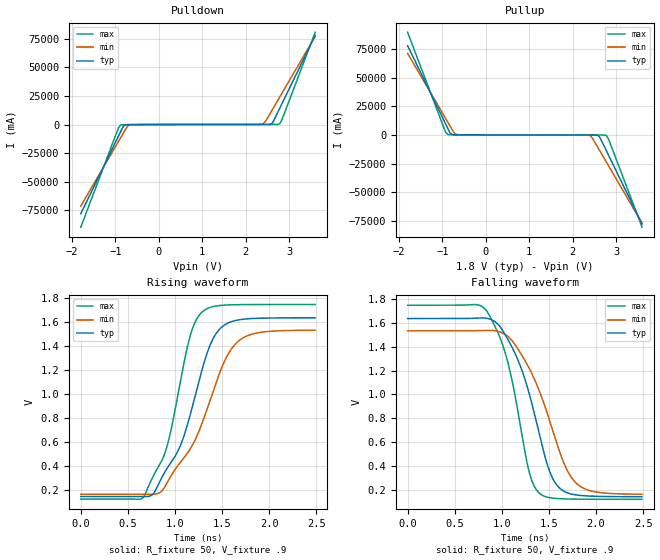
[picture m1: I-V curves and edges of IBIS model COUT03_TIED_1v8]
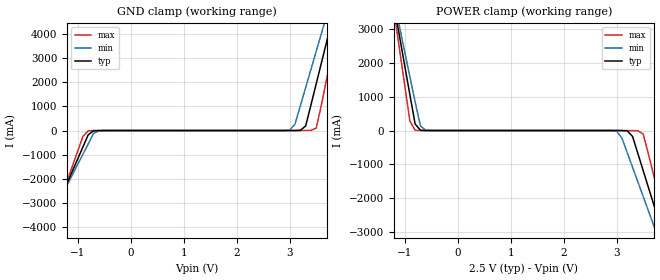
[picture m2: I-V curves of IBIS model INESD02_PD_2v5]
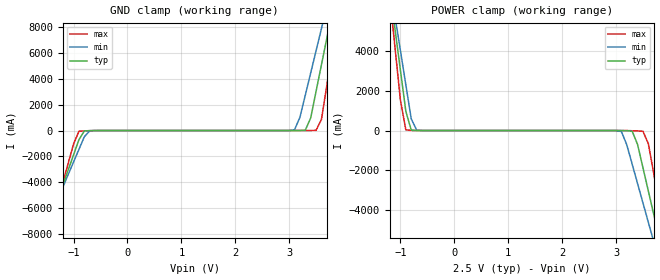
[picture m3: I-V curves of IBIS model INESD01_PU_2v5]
|   This file is an IBIS representation of the   |
|   Integrated Devices Technology, Inc.   |
|   ICS87016   |
|   LOW SKEW, 1-TO-16 LVCMOS/LVTTL CLOCK GENERATOR   |
[IBIS Ver]   4.1
[File name]   87016.ibs
[File Rev]   1.0
[Date]   13 Apr 2009 | Last modified
|   Jan 09 2003 | Generated
[Source]   Originated at Integrated Devices Technology, Inc.
[Disclaimer]
IDT hereby grants the user of this IBIS model a non-exclusive,
nontransferable license to use this IBIS model under the following terms.
Before using this IBIS model, the user should read this license.
If the user does not accept these terms,  the IBIS model should be
returned to IDT within 30 days.
   The user is granted this license only to use the IBIS model and
is not granted rights to sell, load, rent, lease or license the IBIS
model in whole or in part, or in modified form to anyone other than
user. User may modify the IBIS model to suit its specific
applications but rights to derivative works and such modifications
shall belong to IDT.
   This IBIS model is provided on an "AS IS" basis and IDT makes
absolutely no warranty with respect to the information contained
herein. IDT DISCLAIMS AND CUSTOMER WAIVES ALL WARRANTIES, EXPRESS
OR IMPLIED, INCLUDING WARRANTIES OF MERCHANTABILITY OR FITNESS FOR
A PARTICULAR PURPOSE. The entire risk as to quality and performance
is with the Customer. ACCORDINGLY, IN NO EVENT SHALL THE COMPANY BE
LIABLE FOR ANY DAMAGES, WHETHER IN CONTRACT OR TORT,INCLUDING ANY
LOST PROFITS OR OTHER INCIDENTAL, CONSEQUENTIAL, EXEMPLARY, OR
PUNITIVE DAMAGES ARISING OUT OF THE USE OR APPLICATION OF THE IBIS
model provided in this package. Further, IDT reserves the right to
make changes without notice to any product herein to improve
reliability, function, or design. IDT does not convey any license
under patent rights or any other intellectual property rights,
including those of third parties.
   IDT is not obligated to provide maintenance or support
for the licensed IBIS model.
[Copyright]   Copyright 2003 by Integrated Devices Technology, Inc.
[Component]   ICS87016
[Manufacturer] Integrated Devices Technology, Inc.
[Package]
|LQFP48
|lead + wire   typ   min   max
R_pkg   220.4m   212.5m   238m
L_pkg   1.841nH   1.708nH   1.974n
C_pkg   0.316pF   0.2907pF   0.33pF
[Pin] signal_name   model_name  R_pin   L_pin   C_pin
1   VDD   POWER   238m   1.974n   0.338p
2   CLK0   INESD02_PD   225m   1.831n   0.330p
3   DIV_SELA   INESD01_PU   220m   1.781n   0.323p
4   DIV_SELB   INESD01_PU   214m   1.732n   0.312p
5   DIV_SELC   INESD01_PU   214m   1.709n   0.305p
6   DIV_SELD   INESD01_PU   213m   1.708n   0.291p
7   CLK_ENA   INESD01_PU   213m   1.708n   0.291p
8   CLK_ENB   INESD01_PU   214m   1.709n   0.305p
9   CLK_ENC   INESD01_PU   214m   1.732n   0.312p
10   CLK_END   INESD01_PU   220m   1.781n   0.323p
11   nMR/OE   INESD01_PU   225m   1.831n   0.330p
12   GND   GND   238m   1.974n   0.338p
13   QD3   COUT03_TIED  238m   1.974n   0.338p
14   VDDOD   POWER   225m   1.831n   0.330p
15   QD2   COUT03_TIED  220m   1.781n   0.323p
16   GND   GND   214m   1.732n   0.312p
17   QD1   COUT03_TIED  214m   1.709n   0.305p
18   VDDOD   POWER   213m   1.708n   0.291p
19   QD0   COUT03_TIED  213m   1.708n   0.291p
20   GND   GND   214m   1.709n   0.305p
21   QC3   COUT03_TIED  214m   1.732n   0.312p
22   VDDOC   POWER   220m   1.781n   0.323p
23   QC2   COUT03_TIED  225m   1.831n   0.330p
24   GND   GND   238m   1.974n   0.338p
25   QC1   COUT03_TIED  238m   1.974n   0.338p
26   VDDOC   POWER   225m   1.831n   0.330p
27   QC0   COUT03_TIED  220m   1.781n   0.323p
28   GND   GND   214m   1.732n   0.312p
29   QB3   COUT03_TIED  214m   1.709n   0.305p
30   VDDOB   POWER   213m   1.708n   0.291p
31   QB2   COUT03_TIED  213m   1.708n   0.291p
32   GND   GND   214m   1.709n   0.305p
33   QB1   COUT03_TIED  214m   1.732n   0.312p
34   VDDOB   POWER   220m   1.781n   0.323p
35   QB0   COUT03_TIED  225m   1.831n   0.330p
36   GND   GND   238m   1.974n   0.338p
37   QA3   COUT03_TIED  238m   1.974n   0.338p
38   VDDOA   POWER   225m   1.831n   0.330p
39   QA2   COUT03_TIED  220m   1.781n   0.323p
40   GND   GND   214m   1.732n   0.312p
41   QA1   COUT03_TIED  214m   1.709n   0.305p
42   VDDOA   POWER   213m   1.708n   0.291p
43   QA0   COUT03_TIED  213m   1.708n   0.291p
44   GND   GND   214m   1.709n   0.305p
45   CLK_SEL   INESD01_PD   214m   1.732n   0.312p
46   nCLK1   INESD01_PU   220m   1.781n   0.323p
47   CLK1   INESD01_PD   225m   1.831n   0.330p
48   VDD   POWER   238m   1.974n   0.338p
[Diff Pin]  inv_pin  vdiff tdelay_typ tdelay_min  tdelay_max
47   46   0.15   0   0   0
[Model Selector] INESD02_PD
INESD02_PD_2v5  Buffer selection for 2v5
INESD02_PD_3v3  Buffer selection for 3v3
[Model Selector] INESD01_PU
INESD01_PU_2v5  Buffer selection for 2v5
INESD01_PU_3v3  Buffer selection for 3v3
[Model Selector] COUT03_TIED
COUT03_TIED_1v8  Buffer selection for 1v8
COUT03_TIED_2v5  Buffer selection for 2v5
COUT03_TIED_3v3  Buffer selection for 3v3
[Model Selector] INESD01_PD
INESD01_PD_2v5  Buffer selection for 2v5
INESD01_PD_3v3  Buffer selection for 3v3
| Models and submodels in the file (9): COUT03_TIED_1v8 (Output), INESD02_PD_2v5 (Input), INESD01_PU_2v5 (Input), COUT03_TIED_2v5 (Output), INESD01_PD_2v5 (Input), INESD02_PD_3v3 (Input), INESD01_PU_3v3 (Input), COUT03_TIED_3v3 (Output), INESD01_PD_3v3 (Input)
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[Model] COUT03_TIED_1v8
Model_type   Output
Polarity   Non-Inverting
Vmeas = .9
Rref = 50
Cref = 0
Vref = .9
|   typ   min   max
C_comp   2pF   1.5pF   2.5pF
|   typ   min   max
[Voltage range]  1.8V   1.710V   1.890V
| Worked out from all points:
|   slope of the pulldown table from 0 to 0.27 V, typ, clamps not added: 10.3 ohm
|   slope of the pullup table from 0 to 0.27 V, typ, clamps not added: 11.9 ohm
|   rising waveform, R_fixture 50, V_fixture .9: 20-80 % time 370ps typ, 453ps min, 278ps max; typ from 0.143 V to 1.64 V
|   falling waveform, R_fixture 50, V_fixture .9: 20-80 % time 327ps typ, 389ps min, 257ps max; typ from 1.64 V to 0.143 V
[pulldown]
|Voltage   I (typ)   I (min)   I (max)
-1.8V     -77.88A    -71.2A     -89.55A
-927.3mV  -9.821A    -14.52A    -2.535A
-872.7mV  -5.567A    -10.98A    -279.7mA
-818.2mV  -1.447A    -7.441A    -119.4mA
-709.1mV  -98.56mA   -919.5mA   -92.65mA
-654.5mV  -74.81mA   -208.2mA   -85.34mA
2.4V      58.79mA    507.6mA    70.84mA
2.455V    61.02mA    2.637A     70.98mA
2.618V    1.414A     13.25A     71.57mA
2.782V    14.02A     23.86A     493.4mA
2.836V    18.27A     27.4A      4.385A
3.6V      77.78A     76.94A     80.46A
[pullup]
|Voltage   I (typ)   I (min)   I (max)
-1.8V     77.89A     71.2A      89.57A
-927.3mV  9.823A     14.53A     2.543A
-872.7mV  5.569A     10.98A     287mA
-818.2mV  1.45A      7.444A     126.9mA
-709.1mV  101.7mA    922.5mA    99.62mA
-654.5mV  77.73mA    211.3mA    91.37mA
2.4V      -60.59mA   -515mA     -72.08mA
2.455V    -64.65mA   -2.647A    -72.76mA
2.618V    -1.428A    -13.27A    -79.03mA
2.782V    -14.05A    -23.89A    -515mA
2.836V    -18.3A     -27.43A    -4.411A
3.6V      -77.85A    -77.01A    -80.54A
[Ramp]
|   typ   min   max
dV/dt_r   1.195/0.568n   1.097/0.672n   1.302/0.454n
dV/dt_f   1.198/0.499n   1.099/0.587n   1.305/0.4n
[Rising Waveform]
R_fixture = 50
V_fixture = .9
V_fixture_max = .945
V_fixture_min = .855
C_fixture = 0.0p
| Time   typ   min   max
0s        142.8mV    161.8mV    121.5mV
669.8ps   141.6mV    161.9mV    141.9mV
771.9ps   167.8mV    161.3mV    317mV
901.4ps   358.7mV    236.1mV    524.7mV
1.043ns   542.1mV    414.8mV    1.045V
1.17ns    851.2mV    551.4mV    1.508V
1.295ns   1.223V     771mV      1.689V
1.449ns   1.518V     1.122V     1.736V
1.678ns   1.619V     1.444V     1.746V
2.488ns   1.636V     1.533V     1.747V
[Falling Waveform]
R_fixture = 50
V_fixture = .9
V_fixture_max = .945
V_fixture_min = .855
C_fixture = 0.0p
| Time   typ   min   max
0s        1.636V     1.533V     1.747V
844.1ps   1.637V     1.538V     1.693V
1.021ns   1.52V      1.509V     1.386V
1.15ns    1.326V     1.405V     945.8mV
1.287ns   1.015V     1.223V     360mV
1.402ns   652.9mV    1.021V     170.3mV
1.559ns   269.5mV    650.9mV    130mV
1.673ns   183.5mV    397.7mV    124.9mV
1.783ns   159mV      262.2mV    123.1mV
2.488ns   143.1mV    163.6mV    121.5mV
[Model] INESD02_PD_2v5
Model_type   Input
Polarity   Non-Inverting
Vinl = 1.4V
Vinh = 1.85V
|   typ   min   max
C_comp   2pF   1.5pF   2.5pF
|   typ   min   max
[Voltage range]  2.5V   2.375V   2.625V
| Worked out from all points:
|   GND clamp passes 1 mA (typ) near -0.55 V on its own axis
|   POWER clamp passes 1 mA (typ) near -0.60 V on its own axis
[GND_clamp]
|Voltage I(typ)   I(min)   I(max)
-2.5V     -8.775A    -7.892A    -10.18A
-1.6V     -4.218A    -4.001A    -4.586A
-900mV    -678.5mA   -979.3mA   -237.6mA
-800mV    -173.9mA   -548.7mA   -10.83mA
-600mV    -1.629mA   -8.74mA    -911.1uA
3V        133.3uA    17.16mA    56.6uA
3.1V      660.9uA    273.5mA    60.87uA
3.3V      191.6mA    1.785A     327.9uA
3.5V      1.949A     3.298A     103.6mA
3.7V      3.723A     4.812A     2.189A
3.9V      5.498A     6.327A     4.369A
5V        15.27A     14.67A     16.38A
[POWER_clamp]
|Voltage   I(typ)   I(min)   I(max)
-2.5V     15.27A     13.72A     17.74A
-1.2V     3.723A     3.866A     3.551A
-1.1V     2.836A     3.109A     2.461A
-900mV    1.063A     1.596A     283.3mA
-800mV    191.6mA    840.1mA    6.189mA
-600mV    660.9uA    8.845mA    114.2uA
3V        -338.1uA   -16.36mA   -12.68uA
3.4V      -678.5mA   -1.518A    -7.183mA
3.5V      -1.183A    -1.95A     -99.52mA
3.7V      -2.195A    -2.813A    -1.324A
4V        -3.712A    -4.109A    -3.188A
5V        -8.775A    -8.432A    -9.404A
[Model] INESD01_PU_2v5
Model_type   Input
Polarity   Non-Inverting
Vinl = 1.4V
Vinh = 1.85V
|   typ   min   max
C_comp   2pF   1.5pF   2.5pF
|   typ   min   max
[Voltage range]  2.5V   2.375V   2.625V
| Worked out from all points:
|   GND clamp passes 1 mA (typ) near -0.54 V on its own axis
|   POWER clamp passes 1 mA (typ) near -0.66 V on its own axis
[GND_clamp]
|Voltage   I(typ)   I(min)   I(max)
-2.5V     -19.6A     -17.18A    -23.67A
-1.6V     -8.969A    -8.332A    -10.1A
-1.5V     -7.788A    -7.349A    -8.588A
-900mV    -707.1mA   -1.46A     -57.43mA
-700mV    -7.027mA   -24.05mA   -13.28mA
3.1V      199.2uA    53.94mA    11.78uA
3.3V      28.4mA     2.748A     652.4uA
3.5V      3.045A     6.192A     15.72mA
3.6V      5.115A     7.914A     872.4mA
3.7V      7.185A     9.638A     3.52A
3.9V      11.33A     13.09A     8.818A
5V        34.14A     32.07A     37.99A
[POWER_clamp]
|Voltage   I(typ)   I(min)   I(max)
-1.5V     9.257A     9.207A     9.48A
-1.2V     7.185A     7.484A     6.83A
-1.1V     5.115A     5.761A     4.182A
-900mV    976.9mA    2.318A     34.23mA
-700mV    1.582mA    24.31mA    1.044mA
3.1V      -2.107mA   -51.03mA   -534.5uA
3.3V      -35.62mA   -1.705A    -10.86mA
3.5V      -1.886A    -3.666A    -39.41mA
3.6V      -3.066A    -4.647A    -666.9mA
3.8V      -5.426A    -6.612A    -3.684A
3.9V      -6.607A    -7.595A    -5.193A
5V        -19.6A     -18.41A    -21.79A
